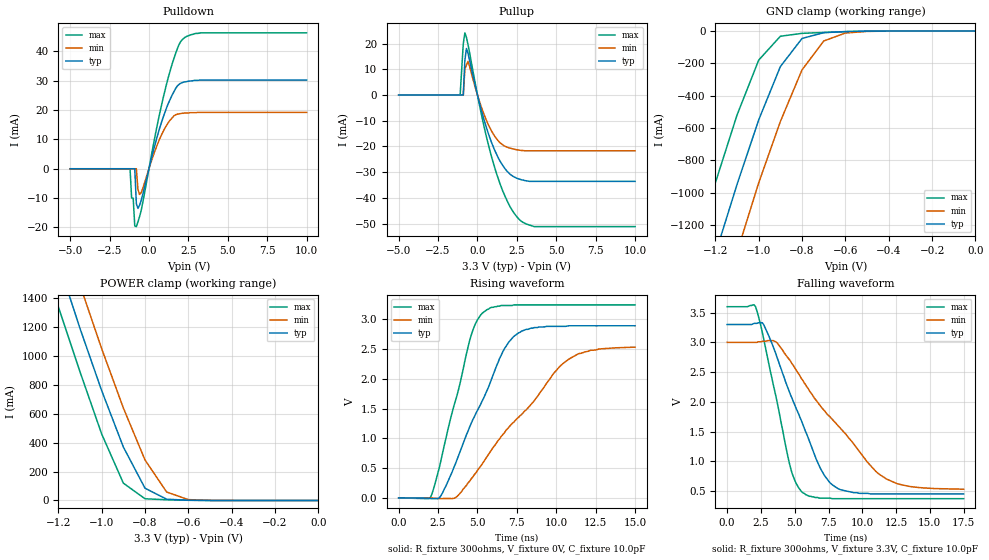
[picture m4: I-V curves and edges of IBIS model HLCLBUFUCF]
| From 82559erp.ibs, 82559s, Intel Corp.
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[Model]   HLCLBUFUCF
Model_type   I/O
Vinl  =   0.8V   | note : D101S spec
Vinh  =   2V   | note : D101S spec
|variable   typ   min  max
C_comp   2.96pF   NA   NA
| note : on die power/gnd supply distribution R/L/C
|   are not included in the simulation
|variable   typ   min   max
[Voltage range]   3.3V   3.0V   3.6V
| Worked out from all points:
|   slope of the pulldown table from 0 to 0.495 V, typ, clamps not added: 47.6 ohm
|   slope of the pullup table from 0 to 0.495 V, typ, clamps not added: 43.8 ohm
|   GND clamp passes 1 mA (typ) near -0.50 V on its own axis
|   POWER clamp passes 1 mA (typ) near -0.55 V on its own axis
|   rising waveform, R_fixture 300ohms, V_fixture 0V, C_fixture 10.0pF: 20-80 % time 2.75ns typ, 4.54ns min, 1.76ns max; typ from 0 V to 2.89 V
|   falling waveform, R_fixture 300ohms, V_fixture 3.3V, C_fixture 10.0pF: 20-80 % time 2.9ns typ, 5.07ns min, 1.76ns max; typ from 3.3 V to 0.45 V
| note : all DC corves are with 0.2 OHM res. series to the PAD.
[GND_clamp]
| Voltage   I(typ)   I(min)   I(max)
-5V       -19.9A     -20.3A     -19.5A
-1.3V     -1.83A     -2.26A     -1.39A
-1.2V     -1.38A     -1.81A     -940mA
-1.1V     -950mA     -1.37A     -520mA
-1V       -550mA     -940mA     -180mA
-900mV    -220mA     -560mA     -32.3mA
-800mV    -45.9mA    -240mA     -14.4mA
-700mV    -10.3mA    -61.7mA    -8.98mA
-600mV    -3.4mA     -12.4mA    -4.05mA
-500mV    -950uA     -2.36mA    -1.01mA
0V        0A         0A         0A
[PullDown]
|Voltage   I(typ)   I(min)   I(max)
-5V       0A         0A         0A
-1.2V     0A         0A         0A
-1.1V     0A         0A         -10mA
-1V       0A         0A         -10mA
-900mV    0A         0A         -19.5mA
-800mV    -11.9mA    0A         -19.7mA
-700mV    -13.5mA    -7mA       -18.1mA
-500mV    -10.9mA    -8.22mA    -14.4mA
900mV     17.5mA     12.7mA     24.1mA
1.5V      25.4mA     17.5mA     36.2mA
2.1V      29.3mA     18.9mA     43.9mA
10V       30.2mA     19.2mA     46.3mA
[POWER_clamp]
| Voltage  I(typ)   I(min)   I(max)
-5V       20.3A      20.5A      20A
-1.3V     2.11A      2.41A      1.81A
-1.2V     1.65A      1.94A      1.34A
-1.1V     1.19A      1.49A      890mA
-1V       760mA      1.05A      460mA
-900mV    370mA      640mA      120mA
-800mV    84.8mA     280mA      11.9mA
-700mV    8.82mA     58.3mA     4.9mA
-600mV    1.74mA     5.95mA     1.41mA
-500mV    290uA      690uA      150uA
0V        1.33nA     19.2nA     440pA
[PullUp]
| Voltage  I(typ)   I(min)   I(max)
-5V       0A         0A         0A
-1.1V     0A         0A         0A
-900mV    0A         0A         20mA
-800mV    13.5mA     10mA       24.2mA
-700mV    18.1mA     11.7mA     22.4mA
-600mV    16.2mA     13.1mA     19.6mA
200mV     -4.87mA    -3.87mA    -6.11mA
900mV     -18.6mA    -14.1mA    -24.2mA
1.6V      -27.4mA    -19.4mA    -37.3mA
2.6V      -32.6mA    -21.4mA    -48.1mA
3.6V      -33.6mA    -21.7mA    -51.2mA
10V       -33.6mA    -21.7mA    -51.2mA
[Ramp]
|Variable   typ   min   max
dV/dt_r   1.77/2.8n   1.50/4.5n   1.99/1.8n
dV/dt_f   1.71/2.9n   1.49/5.1n   1.88/1.7n
R_load  = 300ohms
[Rising Waveform]
|   note : pad parasitics are not incloded
R_fixture   = 300ohms
V_fixture   = 0V
C_fixture   = 10.0pF
|Time   typ(V)   min(V)   max(V)
0s        820pV      19.34nV    330pV
2.1ns     -11.91mV   -1.05mV    57.76mV
2.8ns     93.48mV    -10.95mV   770mV
3.6ns     570mV      3.32mV     1.63V
4.5ns     1.19V      280mV      2.64V
5.3ns     1.63V      570mV      3.1V
6.7ns     2.5V       1.09V      3.23V
7.8ns     2.8V       1.4V       3.24V
10.8ns    2.89V      2.33V      3.24V
15ns      2.89V      2.53V      3.24V
[Falling Waveform]
|   note : pad parasitics are not incloded
R_fixture   = 300ohms
V_fixture   = 3.3V
V_fixture_min   = 3.0V
V_fixture_max   = 3.6V
C_fixture   = 10.0pF
|Time   typ   min   max
0s        3.3V       3V         3.6V
2.1ns     3.32V      3V         3.6V
2.7ns     3.3V       3.02V      3.06V
3.6ns     2.81V      3.01V      2.1V
4.7ns     2.11V      2.68V      880mV
5.6ns     1.62V      2.36V      470mV
7.2ns     760mV      1.85V      380mV
8.4ns     520mV      1.55V      370mV
11.8ns    450mV      700mV      370mV
17.5ns    450mV      530mV      370mV
